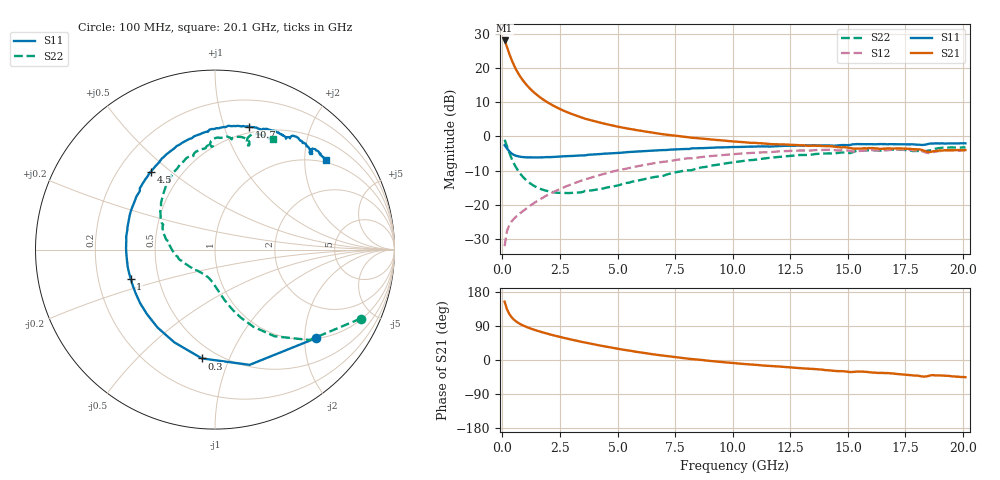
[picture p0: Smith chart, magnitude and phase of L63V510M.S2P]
!  Infineon Technologies AG
! BFR380L3 , PF131585-7, No.6, Th 09.10.01, soldered on pcb-board, measured with PP GSG850
!  Vce=3.5 V,  Ic=10.0 mA
! Common Emitter S-Parameters:  15. November 2001
#  GHz  S  MA  R  50
! f  S11  S21  S12  S22
! GHz  Mag  Ang  Mag  Ang  Mag  Ang  Mag  Ang
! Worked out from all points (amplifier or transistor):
!   201 points, 100 MHz to 20.1 GHz, reference 50 ohm
!   highest |S21| = 28.0 dB at 100 MHz (marker M1)
!   |S21| within 3 dB of that: start of sweep to 258.1 MHz
!   unconditionally stable (mu >= 1): 1.843 GHz to 4.481 GHz
!   at 3.4 GHz: K = 1.03, MAG = 8.3 dB, |S12| = -12.9 dB
!   at 10.1 GHz: K = 0.95, MSG = 1.8 dB, |S12| = -5.1 dB
!   at 20.1 GHz: K = 0.99, MSG = 0.1 dB, |S12| = -4.0 dB
!   S11 on the Smith chart (normalised r, x): 100 MHz: 1.01, -2.26; 300 MHz: 0.41, -0.80; 1 GHz: 0.34, -0.15; 4.5 GHz: 0.34, +0.43; 10.7 GHz: 0.44, +1.21; 20.1 GHz: 0.94, +2.54
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0.1  0.7473 -41.4  25.13 153.8  0.02516 70.9  0.8976 -25.4
0.2  0.6705 -73.3  20.29 134.5  0.04125 58.5  0.7291 -43.7
0.3  0.6107 -96.8  16.19 121.8  0.051 52.4  0.5857 -55.5
0.4  0.5645 -113.6  13.21 113.0  0.05742 49.5  0.481 -63.5
0.5  0.5396 -126.3  11.04 106.6  0.0629 48.9  0.4067 -69.1
0.6  0.5228 -136.2  9.432 101.7  0.06777 49.2  0.3528 -73.4
0.7  0.5132 -144.2  8.234 97.6  0.07249 49.8  0.3119 -76.8
0.8  0.505 -150.7  7.289 94.1  0.07733 50.8  0.2806 -79.8
1  0.4968 -161.0  5.93 88.4  0.08722 52.5  0.237 -84.6
1.2  0.4958 -168.8  4.994 83.6  0.09758 54.1  0.2086 -88.9
1.4  0.4941 -175.4  4.32 79.5  0.1084 55.3  0.1889 -92.8
1.6  0.4956 178.9  3.808 75.6  0.1194 56.2  0.1753 -96.6
1.9  0.5002 171.6  3.244 70.3  0.1363 56.8  0.1621 -102.2
2.6  0.5127 157.7  2.429 59.5  0.1773 56.5  0.1502 -115.9
3.5  0.5294 143.0  1.863 47.1  0.2314 53.7  0.1556 -132.3
4.5  0.5622 129.5  1.518 35.3  0.291 49.1  0.1785 -152.2
6.8  0.6299 104.1  1.099 12.9  0.4198 35.1  0.2622 170.8
10.1  0.7019 78.5  0.8428 -8.4  0.5548 13.5  0.4238 132.8
10.7  0.7105 74.6  0.8115 -11.4  0.5731 9.5  0.451 126.2
13.5  0.7395 60.4  0.7349 -23.6  0.6285 -8.0  0.5482 102.2
16.8  0.7725 48.2  0.6694 -34.8  0.6353 -24.5  0.6387 79.4
20.1  0.7949 38.7  0.6355 -45.4  0.6277 -38.5  0.6937 62.5
